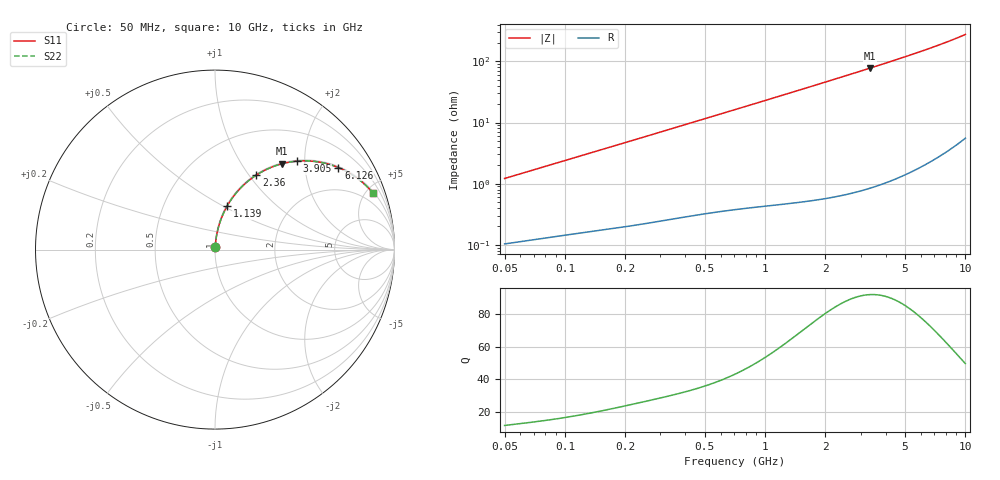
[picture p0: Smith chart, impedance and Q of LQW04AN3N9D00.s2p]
!Murata Part Number: LQW04AN3N9D00
!These Parameters are Measured in Series Mode Connection
!  o--[Z]--o
!Port1  Port2
!  o-------o
!Freq. Start=50[MHz] Stop=10[GHz], 401[Steps]
# Hz S RI R 50
!Freq.(Hz)	S 11(Real)	S 11(Imag)	S 21(Real)	S 21(Imag)	S 12(Real)	S 12(Imag)	S 22(Real)	S 22(Imag)
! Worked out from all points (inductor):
!   401 points, 50 MHz to 10 GHz, reference 50 ohm
!   read as one part in series: L = 3.83 nH near 51.34 MHz
!   highest Q = 92.1 at 3.331 GHz (marker M1), where L = 3.69 nH
!   S11 on the Smith chart (normalised r, x): 50 MHz: 1.00, +0.02; 1.139 GHz: 1.01, +0.52; 2.36 GHz: 1.01, +1.09; 3.905 GHz: 1.02, +1.83; 6.126 GHz: 1.04, +2.98; 10 GHz: 1.11, +5.51
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5e7  0.00118 0.0121  0.9988 -0.0121  0.9988 -0.0121  0.00118 0.0121
1.214486e8  0.00238 0.0286  0.9976 -0.0286  0.9976 -0.0286  0.00238 0.0286
1.956524e8  0.00403 0.0455  0.996 -0.0455  0.996 -0.0455  0.00403 0.0455
2.949953e8  0.00706 0.0679  0.9929 -0.0679  0.9929 -0.0679  0.00706 0.0679
4.689809e8  0.0146 0.1063  0.9854 -0.1063  0.9854 -0.1063  0.0146 0.1063
7.071068e8  0.0291 0.157  0.9709 -0.157  0.9709 -0.157  0.0291 0.157
9.094607e8  0.0452 0.1981  0.9548 -0.1981  0.9548 -0.1981  0.0452 0.1981
1.139142e9  0.0673 0.2421  0.9327 -0.2421  0.9327 -0.2421  0.0673 0.2421
1.408053e9  0.0976 0.2894  0.9024 -0.2894  0.9024 -0.2894  0.0976 0.2894
1.717543e9  0.1374 0.3376  0.8626 -0.3376  0.8626 -0.3376  0.1374 0.3376
2.013439e9  0.1789 0.3771  0.8211 -0.3771  0.8211 -0.3771  0.1789 0.3771
2.360312e9  0.2301 0.4152  0.7699 -0.4152  0.7699 -0.4152  0.2301 0.4152
2.803837e9  0.2972 0.4515  0.7028 -0.4515  0.7028 -0.4515  0.2972 0.4515
3.330706e9  0.3753 0.4788  0.6247 -0.4788  0.6247 -0.4788  0.3753 0.4788
3.904516e9  0.455 0.4925  0.545 -0.4925  0.545 -0.4925  0.455 0.4925
4.171863e9  0.4895 0.4944  0.5105 -0.4944  0.5105 -0.4944  0.4895 0.4944
5.021877e9  0.5872 0.4865  0.4128 -0.4865  0.4128 -0.4865  0.5872 0.4865
6.125686e9  0.6875 0.4571  0.3125 -0.4571  0.3125 -0.4571  0.6875 0.4571
6.993273e9  0.7485 0.4268  0.2515 -0.4268  0.2515 -0.4268  0.7485 0.4268
7.983737e9  0.8029 0.3899  0.1971 -0.3899  0.1971 -0.3899  0.8029 0.3899
9.114482e9  0.8501 0.348  0.1499 -0.348  0.1499 -0.348  0.8501 0.348
1e10  0.8787 0.3166  0.1213 -0.3166  0.1213 -0.3166  0.8787 0.3166
